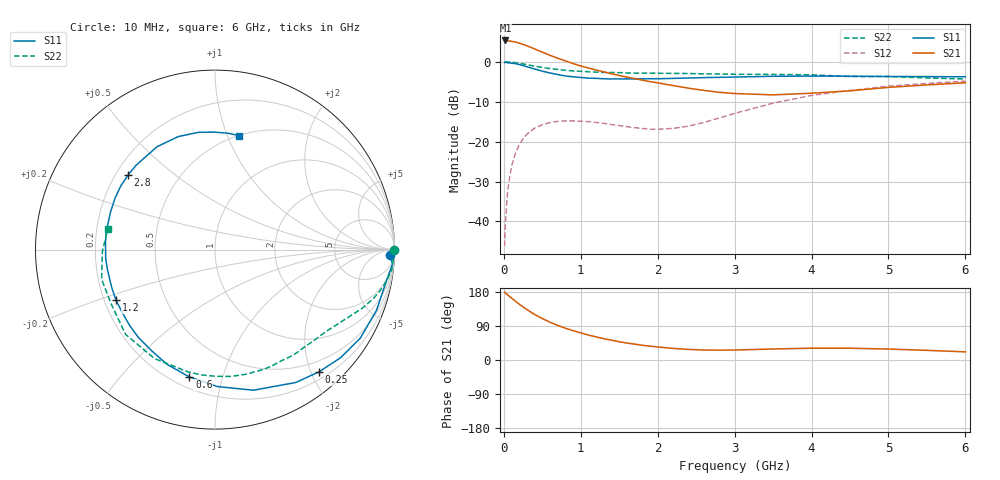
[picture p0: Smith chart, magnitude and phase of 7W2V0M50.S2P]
! Infineon Technologies  Discrete & RF Semiconductors
! BFS17W
! Si NPN RF Bipolar Junction Transistor in SOT323
! VCE = 2 V  IC = 0.5 mA
! Common Emitter S-Parameters:  August  1999
# GHz  S  MA  R  50
!  f  S11  S21  S12  S22
! GHz  MAG  ANG  MAG  ANG  MAG  ANG  MAG  ANG
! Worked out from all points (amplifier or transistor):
!   36 points, 10 MHz to 6 GHz, reference 50 ohm
!   highest |S21| = 5.3 dB at 20 MHz (marker M1)
!   |S21| within 3 dB of that: start of sweep to 508.6 MHz
!   unconditionally stable (mu >= 1): 1.172 GHz to end of sweep
!   at 250 MHz: K = 0.24, MSG = 11.8 dB, |S12| = -19.3 dB
!   at 1.4 GHz: K = 1.19, MAG = 3.7 dB, |S12| = -15.7 dB
!   at 6 GHz: K = 1.11, MAG = -2.2 dB, |S12| = -4.8 dB
!   S11 on the Smith chart (normalised r, x): 10 MHz: 29, -40; 250 MHz: 0.31, -2.13; 600 MHz: 0.26, -0.78; 1.2 GHz: 0.25, -0.23; 2.8 GHz: 0.25, +0.35; 6 GHz: 0.50, +1.10
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0.01  0.9764 -1.9  1.831 179.2  0.0049 86.2  0.9999 -0.2
0.02  0.9919 -4.6  1.85 176.7  0.0095 88.8  0.9983 -1.3
0.05  0.9706 -10.5  1.834 171.5  0.0245 84.0  0.9951 -3.3
0.1  0.9613 -20.6  1.805 163.6  0.0491 77.2  0.9909 -6.6
0.15  0.948 -31.4  1.768 155.1  0.0709 71.0  0.9744 -9.7
0.25  0.8943 -49.6  1.65 140.0  0.1084 59.7  0.9388 -15.2
0.3  0.8665 -58.7  1.588 133.0  0.1239 55.2  0.9206 -17.5
0.4  0.8122 -74.7  1.449 120.2  0.1477 46.4  0.8821 -21.8
0.5  0.7632 -89.0  1.32 109.4  0.1623 39.5  0.849 -25.1
0.6  0.7236 -101.4  1.205 99.7  0.1735 34.0  0.8218 -28.2
0.8  0.6644 -122.3  1.027 84.0  0.1817 25.9  0.7828 -33.9
1.1  0.6236 -146.5  0.837 65.8  0.1779 19.3  0.7499 -42.1
1.2  0.6195 -153.0  0.788 61.0  0.1735 18.1  0.7418 -45.1
1.6  0.6111 -175.6  0.642 44.7  0.1536 19.5  0.725 -56.9
2.2  0.6191 159.8  0.504 30.6  0.1463 38.8  0.7155 -76.1
2.8  0.6383 139.3  0.415 26.0  0.1972 56.0  0.7023 -96.3
3.5  0.658 119.4  0.385 29.1  0.3032 57.6  0.6943 -119.1
4  0.6623 108.0  0.404 31.1  0.379 52.1  0.6865 -136.5
4.5  0.66 97.8  0.433 31.1  0.4369 45.4  0.6531 -152.1
5  0.6545 90.2  0.478 28.9  0.4951 39.0  0.6531 -165.3
5.5  0.6523 83.6  0.513 25.5  0.5356 32.5  0.6277 -179.0
6  0.649 78.2  0.546 21.4  0.5728 26.6  0.6082 169.2
